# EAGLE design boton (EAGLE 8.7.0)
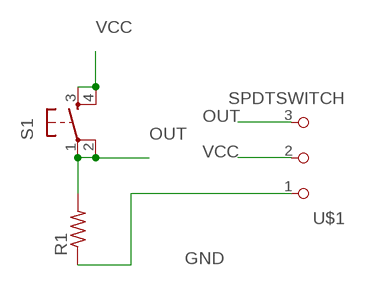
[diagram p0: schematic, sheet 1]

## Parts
R1  RES-US1206FAB  [R1206FAB]
S1  6MM_SWITCH6MM_SWITCH  [6MM_SWITCH]
U$1  SPDTSWITCH  [SPDTSWITCH]

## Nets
GND: R1.1 U$1.1
OUT: R1.2 S1.1(P) S1.2(P1) U$1.3
VCC: S1.3(S) S1.4(S1) U$1.2

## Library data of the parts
R1 = fab:RES-US: Resistor (US Symbol)
S1 = fab:6MM_SWITCH: OMRON SWITCH
U$1 = fab:SPDTSWITCH

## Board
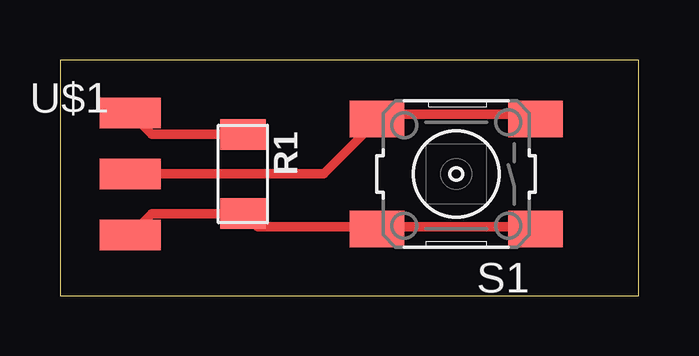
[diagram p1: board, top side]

Size 24.11 x 9.83 mm. Coordinates in mm from the lower left corner, seen from the top.
Outline: 0,0 24.11,0 24.11,9.83 0,9.83 0,0
Copper layers (1*16): Top 0.045mm / dielectric 1.5mm / Bottom 0.045mm
Design rules "default *": minimum track width 0.4mm, minimum drill 0.4mm, track to track 6mil, track to pad 6mil, pad to pad 6mil, via to via 6mil, smd to smd 6mil, copper to edge 40mil, drill to drill 6mil, minimum pad ring 10mil, minimum via ring 8mil, stop-mask expansion 4mil, vias tented up to drill 0mil, thermal gap 10mil

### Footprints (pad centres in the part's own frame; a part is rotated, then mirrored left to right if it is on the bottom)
R1206FAB = smd 1.27 x 1.905: 1 -1.651,0; 2 1.651,0
6MM_SWITCH = smd 2.286 x 1.524: 1 -3.302,2.286; 2 3.302,2.286; 3 -3.302,-2.286; 4 3.302,-2.286
SPDTSWITCH = smd 2.54 x 1.27: 1 0.38,2.54; 2 0.38,0; 3 0.38,-2.54

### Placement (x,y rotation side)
R1  7.62,5.08 270 top
S1  16.51,5.08 180 top
U$1  2.54,5.08 0 top

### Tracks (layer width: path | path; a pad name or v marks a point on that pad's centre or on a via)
GND
  Top 0.4: R1.1 7.4,6.74 3.81,6.74 2.98,7.57 U$1.1
OUT
  Top 0.4: U$1.3 2.98,2.6 3.81,3.43 7.4,3.43 R1.2 7.68,3.43 8.23,2.88 13.2,2.88 S1.2 13.48,2.88 19.56,2.88 S1.1
VCC
  Top 0.4: S1.3 19.56,7.57 13.48,7.57 S1.4 13.2,7.29 10.99,5.08 2.98,5.08 U$1.2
